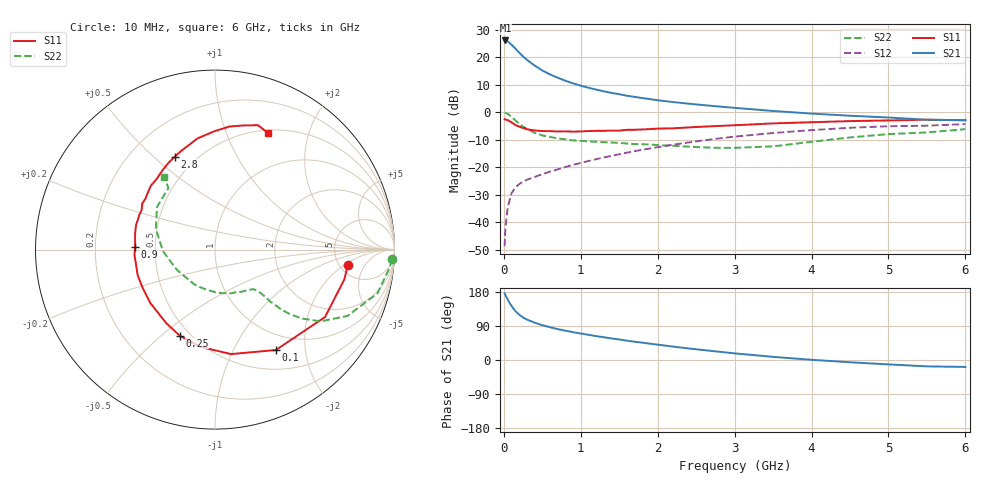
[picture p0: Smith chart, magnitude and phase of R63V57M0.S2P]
! SIEMENS Small Signal Semiconductors
! BFR193
! Si NPN RF Bipolar Junction Transistor in SOT23
! VCE = 3.5 V  IC = 7 mA
! Common Emitter S-Parameters:  May  1996
# GHz  S  MA  R  50
!  f  S11  S21  S12  S22
! GHz  MAG  ANG  MAG  ANG  MAG  ANG  MAG  ANG
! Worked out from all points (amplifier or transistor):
!   36 points, 10 MHz to 6 GHz, reference 50 ohm
!   highest |S21| = 26.1 dB at 20 MHz (marker M1)
!   |S21| within 3 dB of that: start of sweep to 151.1 MHz
!   unconditionally stable (mu >= 1): 821.7 MHz to 1.973 GHz
!   at 250 MHz: K = 0.53, MSG = 22.7 dB, |S12| = -25.2 dB
!   at 1.4 GHz: K = 1.05, MAG = 10.0 dB, |S12| = -15.8 dB
!   at 6 GHz: K = 0.96, MSG = 0.7 dB, |S12| = -4.3 dB
!   lowest NFmin = 1.20 dB at 450 MHz
!   S11 on the Smith chart (normalised r, x): 10 MHz: 5.96, -2.26; 100 MHz: 0.76, -1.49; 250 MHz: 0.44, -0.58; 900 MHz: 0.38, +0.02; 2.8 GHz: 0.39, +0.59; 6 GHz: 0.53, +1.42
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0.01  0.7449 -6.5  20.02 176.0  0.0037 88.2  0.9878 -3.1
0.02  0.7398 -12.9  20.12 171.3  0.0079 83.9  0.9766 -6.2
0.05  0.7191 -31.5  19.41 159.4  0.0186 75.0  0.937 -15.1
0.1  0.6541 -58.8  16.82 142.6  0.0337 64.6  0.8256 -26.6
0.15  0.589 -81.3  14.3 128.9  0.0431 57.4  0.7111 -34.2
0.2  0.5478 -98.5  12.1 119.5  0.0497 54.4  0.6185 -38.4
0.25  0.5182 -112.3  10.27 112.3  0.0551 52.0  0.5487 -40.8
0.3  0.4917 -123.5  8.95 106.7  0.0594 51.3  0.4972 -42.1
0.4  0.4674 -140.4  7.054 98.5  0.0668 52.3  0.4233 -43.2
0.5  0.456 -152.0  5.728 91.8  0.0751 53.4  0.3796 -43.3
0.6  0.454 -161.6  4.863 86.4  0.0836 55.0  0.3554 -43.5
0.7  0.4475 -169.2  4.239 81.5  0.0919 56.3  0.3363 -44.1
0.9  0.4448 177.8  3.348 73.4  0.1109 58.6  0.3085 -45.7
1.1  0.4546 168.1  2.791 66.5  0.1303 59.9  0.2962 -49.1
1.3  0.4607 159.0  2.399 60.0  0.1513 60.3  0.2856 -52.8
1.6  0.4799 147.6  1.998 51.0  0.1847 59.8  0.2708 -60.5
2.2  0.5108 129.4  1.531 35.4  0.2577 55.7  0.2462 -80.6
2.8  0.5646 113.3  1.27 21.8  0.3348 48.7  0.2255 -109.8
3.5  0.6272 98.9  1.056 8.3  0.4195 38.2  0.2405 -152.1
4.5  0.6905 83.3  0.864 -6.0  0.5222 22.5  0.3488 160.7
5.5  0.733 71.0  0.731 -16.8  0.5704 6.2  0.4305 127.0
6  0.7143 65.5  0.718 -18.3  0.6093 1.4  0.4931 125.0
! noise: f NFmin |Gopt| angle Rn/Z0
0.45  1.2  0.24  125  0.12
0.9  1.25  0.36  154  0.11
1.8  2  0.55  -156  0.13
